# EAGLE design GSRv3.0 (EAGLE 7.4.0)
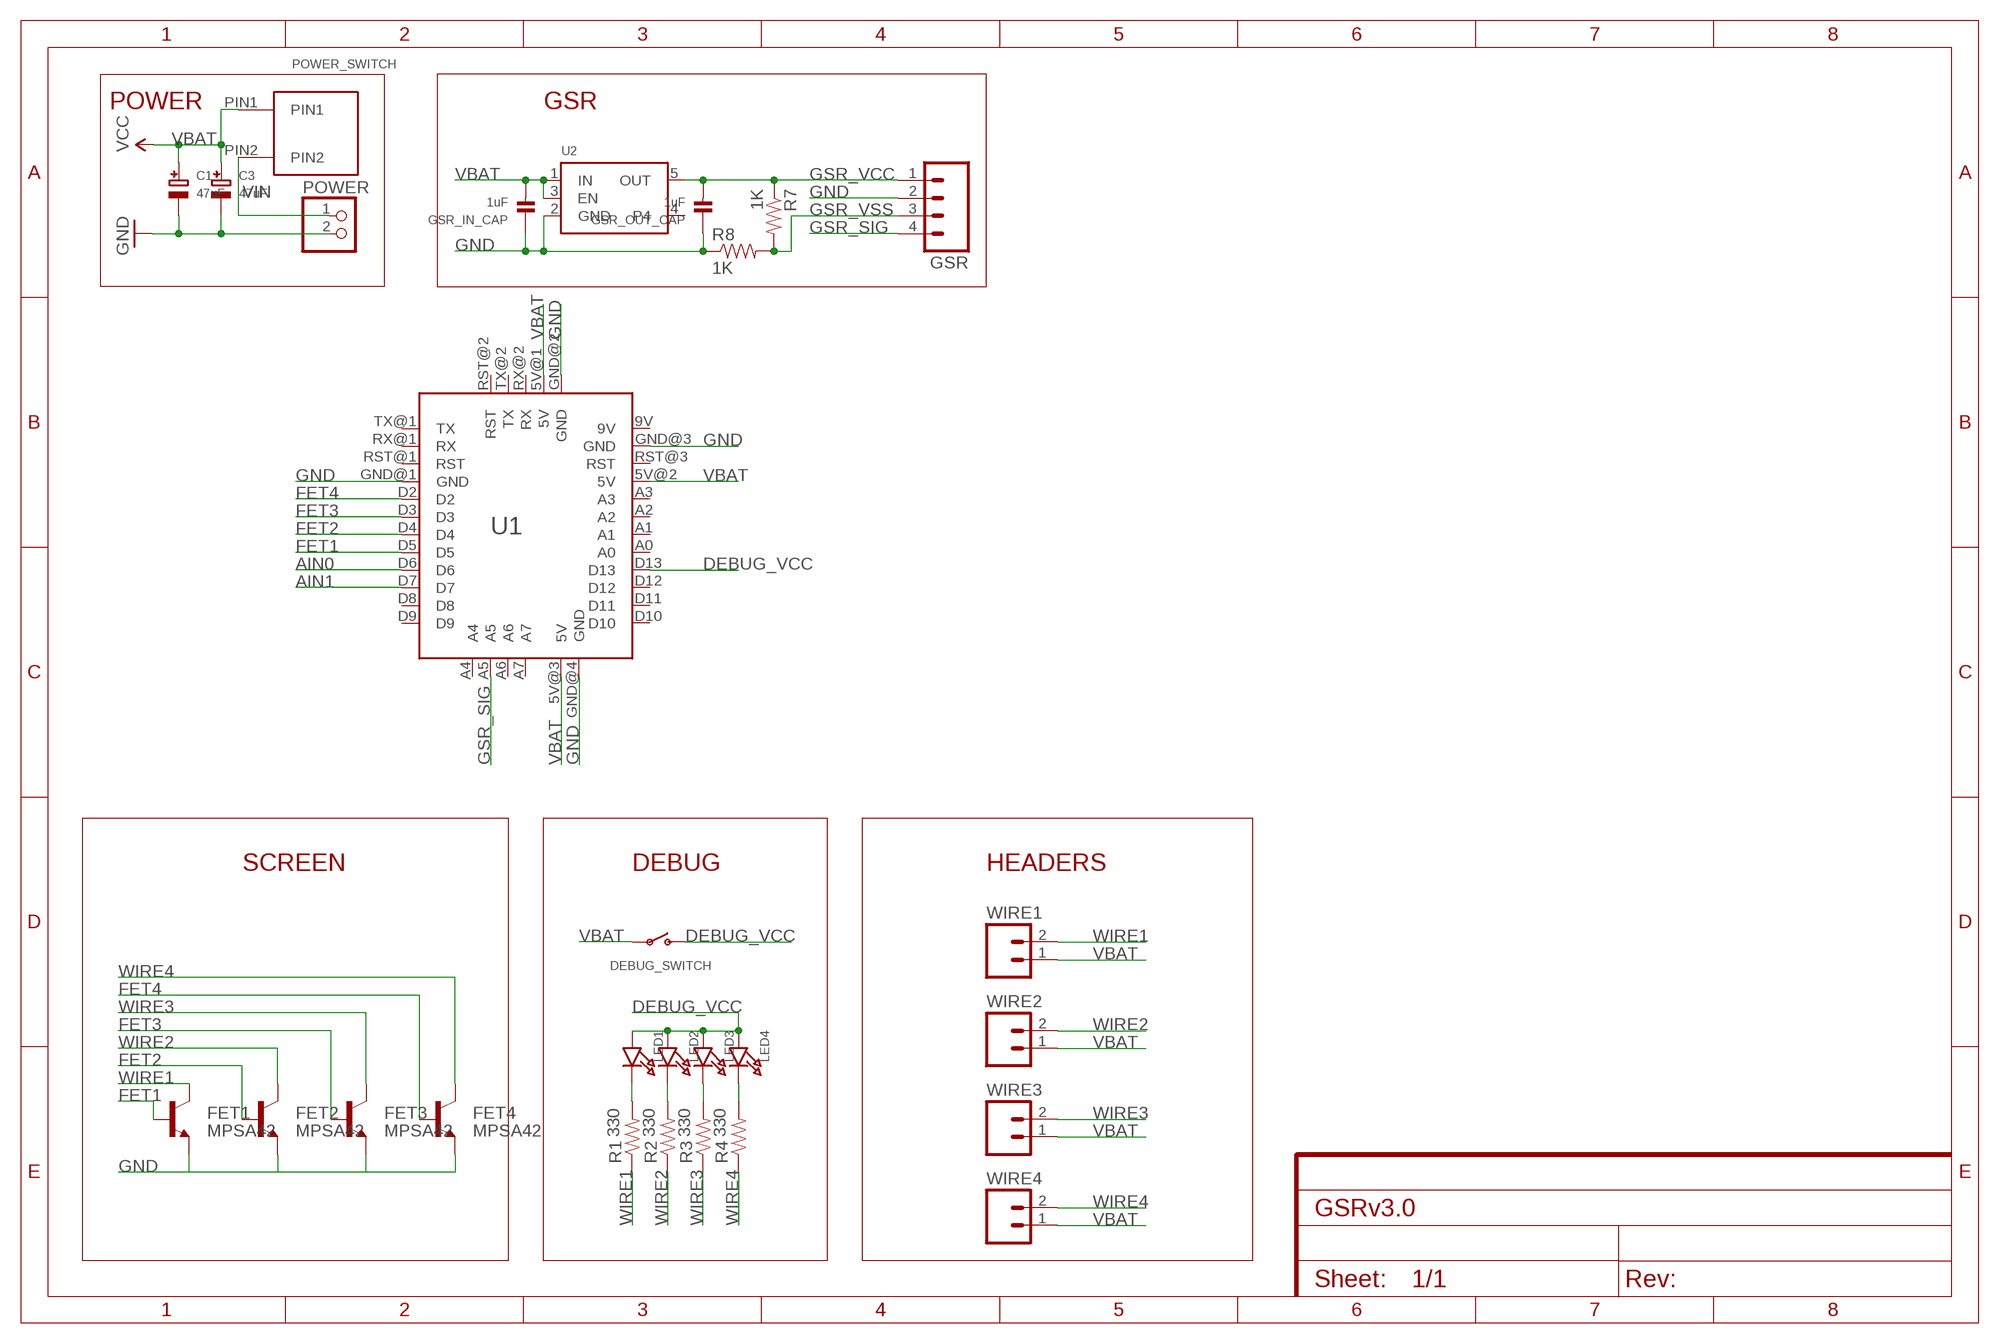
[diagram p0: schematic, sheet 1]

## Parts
C1  47uF  CAP_TANTALUMB/3528_WAVE  [EIA3528-21/B-W]
C3  47uF  CAP_TANTALUMB/3528_WAVE  [EIA3528-21/B-W]
DEBUG_SWITCH  SWITCH_SPST  [SPST_SMT_19192]
FET1  MPSA42  TRANSISTOR_NPNMPSA42  [SOT23-3]
FET2  MPSA42  TRANSISTOR_NPNMPSA42  [SOT23-3]
FET3  MPSA42  TRANSISTOR_NPNMPSA42  [SOT23-3]
FET4  MPSA42  TRANSISTOR_NPNMPSA42  [SOT23-3]
GSR  M04PTH  [1X04]
GSR_IN_CAP  1uF  CAP_CERAMIC0603  [0603]
GSR_OUT_CAP  1uF  CAP_CERAMIC0603  [0603]
LED1  LED0603_NOOUTLINE  [CHIPLED_0603_NOOUTLINE]
LED2  LED0603_NOOUTLINE  [CHIPLED_0603_NOOUTLINE]
LED3  LED0603_NOOUTLINE  [CHIPLED_0603_NOOUTLINE]
LED4  LED0603_NOOUTLINE  [CHIPLED_0603_NOOUTLINE]
POWER  JST_2PIN  [JSTPH2]
POWER_SWITCH  PUSH_BUTTON  [PUSH_BUTTON]
R1  330  RESISTOR0603-RES  [0603-RES]
R2  330  RESISTOR0603-RES  [0603-RES]
R3  330  RESISTOR0603-RES  [0603-RES]
R4  330  RESISTOR0603-RES  [0603-RES]
R7  1K  0OHM-1/10W-5%(0603)  [0603]
R8  1K  0OHM-1/10W-5%(0603)  [0603]
U1  ARDUINO_MINI  [ARDUINO_MINI]
U2  VREG_SOT23-5  [SOT23-5]
WIRE1  M02PTH  [1X02]
WIRE2  M02PTH  [1X02]
WIRE3  M02PTH  [1X02]
WIRE4  M02PTH  [1X02]

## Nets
AIN0: U1.D6
AIN1: U1.D7
DEBUG_VCC: DEBUG_SWITCH.C(S) LED1.A LED2.A LED3.A LED4.A U1.D13
FET1: FET1.1(B) U1.D5
FET2: FET2.1(B) U1.D4
FET3: FET3.1(B) U1.D3
FET4: FET4.1(B) U1.D2
GND: C1.- C3.- FET1.2(E) FET2.2(E) FET3.2(E) FET4.2(E) GSR.2 GSR_IN_CAP.1 GSR_OUT_CAP.1 POWER.2 R8.1 U1.GND@1(GND) U1.GND@2(GND) U1.GND@3(GND) U1.GND@4(GND) U2.2(GND)
GSR_SIG: GSR.4 U1.A5
GSR_VCC: GSR.1 GSR_OUT_CAP.2 R7.1 U2.5(OUT)
GSR_VSS: GSR.3 R7.2 R8.2
N$1: LED1.C R1.2
N$2: LED2.C R2.2
N$3: LED3.C R3.2
N$4: LED4.C R4.2
VBAT: C1.+ C3.+ DEBUG_SWITCH.B(P) GSR_IN_CAP.2 POWER_SWITCH.PIN1 U1.5V@1(5V) U1.5V@2(5V) U1.5V@3(5V) U2.1(IN) U2.3(EN) WIRE1.1 WIRE2.1 WIRE3.1 WIRE4.1 ; supply symbol labelled VCC
VIN: POWER.1 POWER_SWITCH.PIN2
WIRE1: FET1.3(C) R1.1 WIRE1.2
WIRE2: FET2.3(C) R2.1 WIRE2.2
WIRE3: FET3.3(C) R3.1 WIRE3.2
WIRE4: FET4.3(C) R4.1 WIRE4.2
Unconnected: U1.A0 U1.A1 U1.A2 U1.A3 U1.A4 U1.A6 U1.A7 U1.D8 U1.D9 U1.D10 U1.D11 U1.D12 U1.RST@1(RST) U1.RST@2(RST) U1.RST@3(RST) U1.RX@1(RX) U1.RX@2(RX) U1.TX@1(TX) U1.TX@2(TX) U2.4

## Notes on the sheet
- POWER | GSR
- SCREEN | DEBUG | HEADERS

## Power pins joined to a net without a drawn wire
9V: U1.9V

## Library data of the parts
C1 C3 = microbuilder:CAP_TANTALUM: Tantalum Capacitors
DEBUG_SWITCH = microbuilder:SWITCH_SPST: Switch - SPST
FET1-FET4 = SparkFun-DiscreteSemi:TRANSISTOR_NPN: Generic NPN BJT MMBT2222A - TRANS-08049 (SOT-23, 1A 40V) MPSA42 - TRANS-09116 (SOT-23, 500mA 300V) MMBT5088LT1G - TRANS-11160 (SOT-23, 50 mA 30V) BC547 - COM-08928 (TO-92 45V 100mA) (1.Collector 2.Base 3.Emitter) 2N3904 - COM-00521 (TO-92 40V 200mA) (1.Emitter 2.Base 3.Collector) P2N2222A -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; PROD_ID: TRANS-09116
GSR = SparkFun-Connectors:M04: Header 4 Standard 4-pin 0.1" header. Use with straight break away headers (SKU : PRT-00116), right angle break away headers (PRT-00553), swiss pins (PRT-00743), machine pins (PRT-00117), and female headers (PRT-00115). Molex polarized connector foot print use with SKU : PRT-08231 with associated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
GSR_IN_CAP GSR_OUT_CAP = microbuilder:CAP_CERAMIC: Ceramic Capacitors
LED1-LED4 = microbuilder:LED: LED
POWER = microbuilder:JST_2PIN: JST 2-Pin Right-Angle Connector
POWER_SWITCH = myParts:PUSH_BUTTON
R1-R4 = SparkFun-Passives:RESISTOR: Resistor
R7 R8 = SparkFun-Resistors:0OHM-1/10W-5%(0603): RES-08609; PROD_ID: RES-08609; VALUE: 0
U1 = myParts:ARDUINO_MINI: Arduino Mini V5 Footprint
U2 = microbuilder:VREG_SOT23-5: SOT23-5 Fixed Voltage Regulators To better organise some of the SOT23-5 fixed voltage regulators in this library, this new part was created. Part Current Out V Out V In V Dropout Digikey Part No. ADP121 150mA 3.3V 3.4-5.5V 0.09V @ 150mA ADP121-AUJZ33R7CT-ND ADP121 150mA 3.0V 3.1-5.5V 0.09V @ 150mA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
WIRE1-WIRE4 = SparkFun-Connectors:M02: Standard 2-pin 0.1" header. Use with

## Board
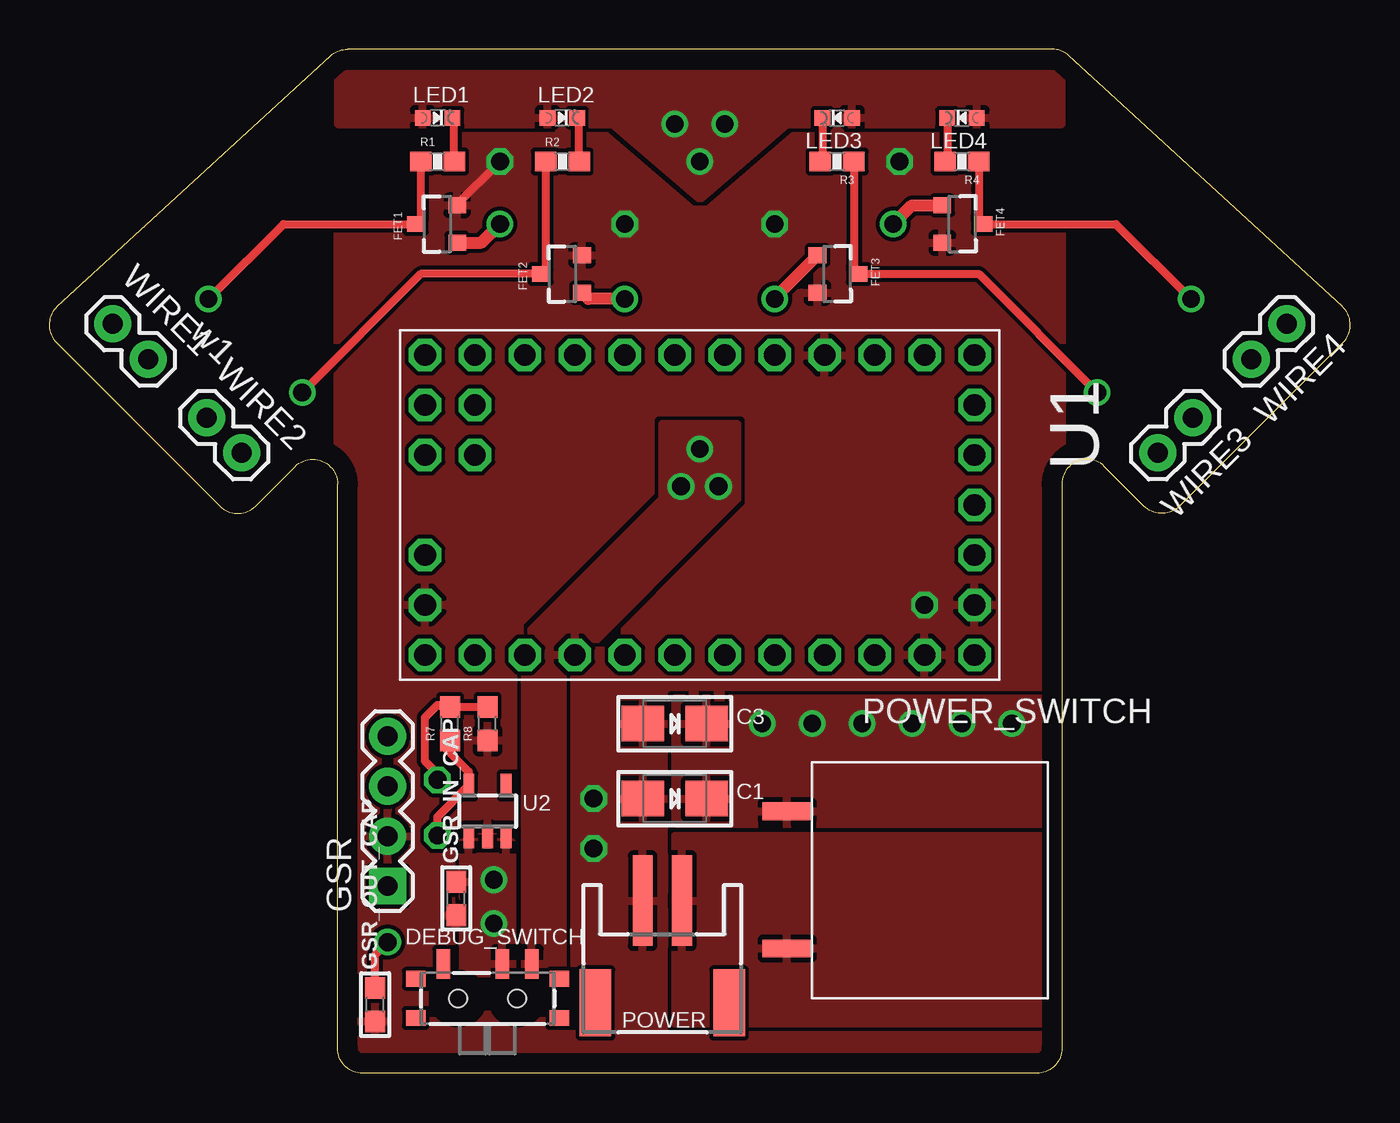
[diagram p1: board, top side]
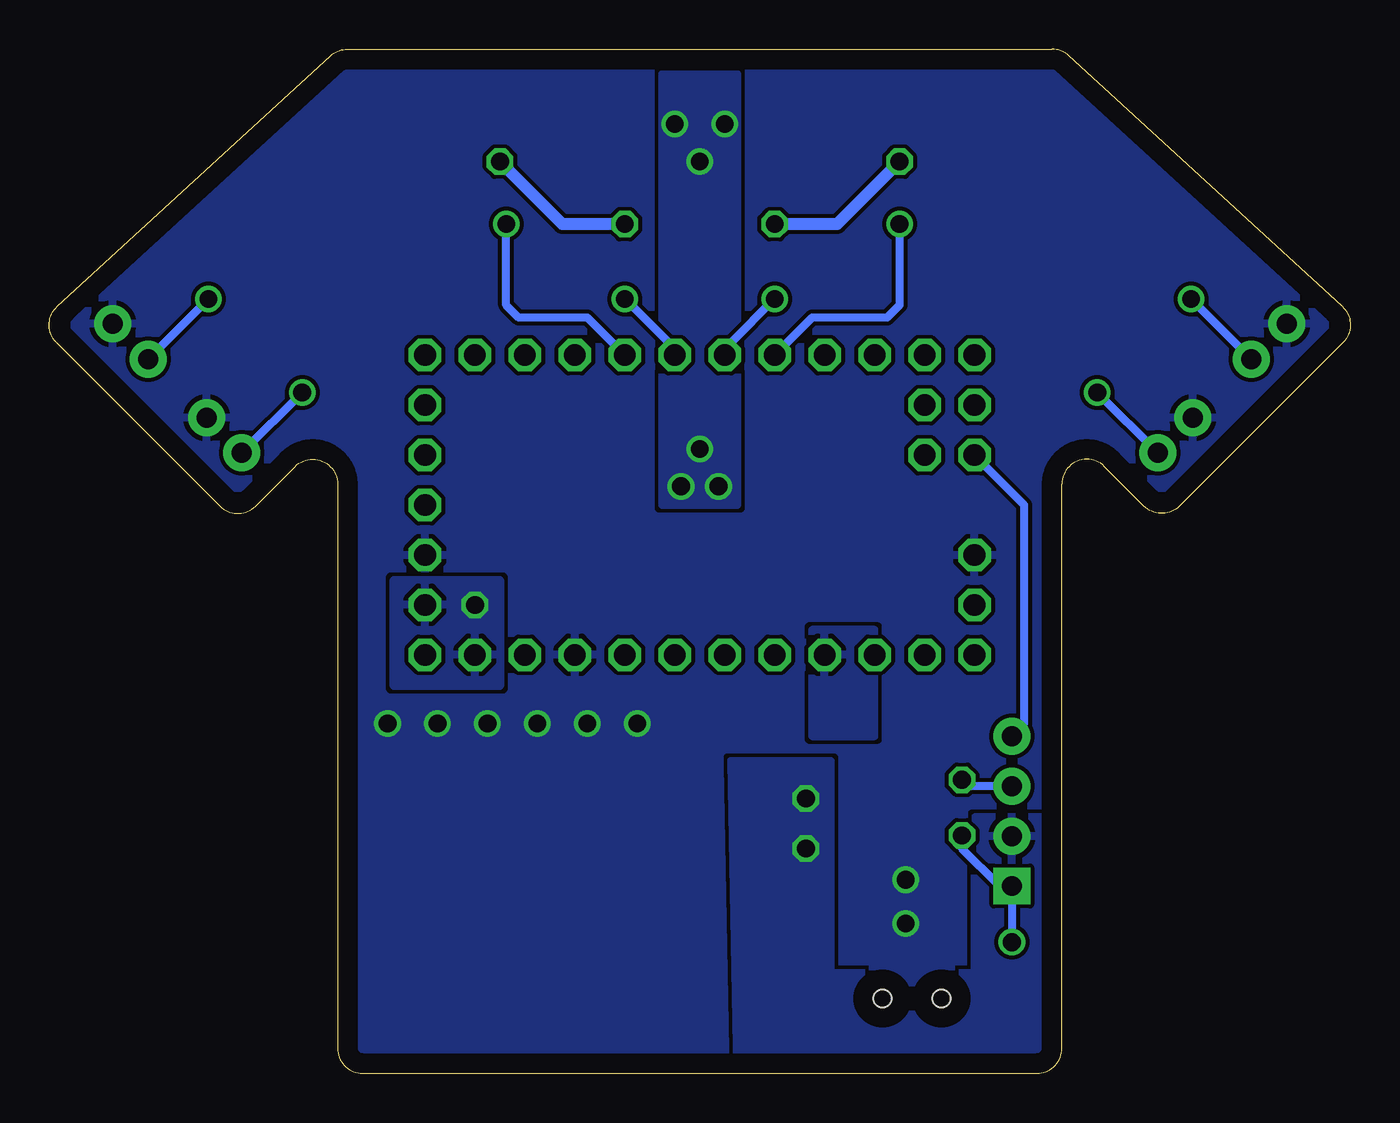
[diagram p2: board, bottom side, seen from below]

Size 66.18 x 52.07 mm. Coordinates in mm from the lower left corner, seen from the top.
Outline: 0.41,39 14.31,51.74 arc-43 15.17,52.07 51.01,52.07 arc-43 51.87,51.74 65.77,39 arc-92 65.81,37.16 57.48,28.84 arc-90 55.69,28.84 53.67,30.85 arc135 51.5,29.95 51.5,1.27 arc-90 50.23,0 15.94,0 arc-90 14.67,1.27 14.67,29.95 arc135 12.51,30.85 10.49,28.84 arc-90 8.7,28.84 0.37,37.16 arc-92 0.41,39
Copper layers (1*16): Top 0.035mm / dielectric 1.5mm / Bottom 0.035mm
Design rules "default": minimum track width 10mil, minimum drill 24mil, track to track 8mil, track to pad 8mil, pad to pad 8mil, via to via 8mil, smd to smd 8mil, copper to edge 40mil, drill to drill 8mil, minimum pad ring 10mil, minimum via ring 8mil, stop-mask expansion 4mil, vias tented up to drill 0mil, thermal gap 10mil

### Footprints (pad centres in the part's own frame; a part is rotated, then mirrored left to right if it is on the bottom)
EIA3528-21/B-W = smd 2.15 x 1.8: + 1.625,0; - -1.625,0
SPST_SMT_19192 = smd 0.7 x 1.5: A -2.25,1.75; B 0.75,1.75; C 2.25,1.75 | smd 1 x 0.8: GND1 -3.65,1; GND2 -3.65,-1; GND3 3.65,1; GND4 3.65,-1 | hole 0.9: -1.5,0; 1.5,0
SOT23-3 = smd 0.8 x 0.9: 1 -0.95,-1; 2 0.95,-1; 3 0,1.1
1X04 = drill 1.016 pad 1.88 square: 1 0,0 | drill 1.016 pad 1.88: 2 2.54,0; 3 5.08,0; 4 7.62,0
0603 = smd 1.1 x 1: 1 -0.85,0; 2 0.85,0
CHIPLED_0603_NOOUTLINE = smd 0.8 x 0.8: A 0,-0.75; C 0,0.75
JSTPH2 = smd 1 x 4.6: 1 -1,-3.7; 2 1,-3.7 | smd 1.6 x 3.4: NC1 -3.4,1.5; NC2 3.4,1.5
PUSH_BUTTON = smd 2.5 x 0.9: PIN1 -13.97,-0.644; PIN2 -13.97,-7.62
0603-RES = smd 1.1 x 1: 1 -0.85,0; 2 0.85,0
ARDUINO_MINI = drill 1.1 octagon: 5V@1 2.54,15.24; 5V@2 7.62,7.62; 5V@3 2.54,-12.7; 9V 7.62,15.24; A0 7.62,-2.54; A1 7.62,0; A2 7.62,2.54; A3 7.62,5.08; A4 -5.08,-12.7; A5 -2.54,-12.7; A6 -5.08,-10.16; A7 -2.54,-10.16; D2 -7.62,5.08; D3 -7.62,2.54; D4 -7.62,0; D5 -7.62,-2.54; D6 -7.62,-5.08; D7 -7.62,-7.62; D8 -7.62,-10.16; D9 -7.62,-12.7; D10 7.62,-12.7; D11 7.62,-10.16; D12 7.62,-7.62; D13 7.62,-5.08; GND@1 -7.62,7.62; GND@2 5.08,15.24; GND@3 7.62,12.7; GND@4 5.08,-12.7; RST@1 -7.62,10.16; RST@2 -5.08,15.24; RST@3 7.62,10.16; RX@1 -7.62,12.7; RX@2 0,15.24; TX@1 -7.62,15.24; TX@2 -2.54,15.24
SOT23-5 = smd 0.55 x 1.2: 1 -0.95,-1.3; 2 0,-1.3; 3 0.95,-1.3; 4 0.95,1.3; 5 -0.95,1.3
1X02 = drill 1.016 pad 1.88: 1 0,0; 2 2.54,0

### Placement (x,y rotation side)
C1  31.82,13.97 0 top
C3  31.82,17.78 0 top
DEBUG_SWITCH  22.29,3.81 0 top
FET1  19.75,43.18 90 top
FET2  26.1,40.64 90 top
FET3  40.07,40.64 270 top
FET4  46.42,43.18 270 top
GSR  17.21,9.53 90 top
GSR_IN_CAP  20.71,8.89 90 top
GSR_OUT_CAP  16.58,3.49 90 top
LED1  19.75,48.58 270 top
LED2  26.1,48.58 270 top
LED3  40.07,48.58 90 top
LED4  46.42,48.58 90 top
POWER  31.18,5.08 180 top
POWER_SWITCH  51.5,13.97 0 top
R1  19.75,46.35 0 top
R2  26.1,46.35 0 top
R3  40.07,46.35 180 top
R4  46.42,46.35 180 top
R7  20.39,17.78 90 top
R8  22.29,17.78 90 top
U1  31.82,28.89 270 top
U2  22.29,13.34 0 top
WIRE1  3.24,38.1 315 top
WIRE2  8.01,33.34 315 top
WIRE3  58.17,33.34 225 top
WIRE4  62.93,38.1 225 top

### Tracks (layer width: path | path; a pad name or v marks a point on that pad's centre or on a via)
DEBUG_VCC  (via drill 0.9)
  other vias: 33.09,31.75 32.14,29.84 34.04,29.84 33.09,46.35 31.82,48.26 34.36,48.26
  pour Bottom: 34.99,28.89 34.99,50.8 31.18,50.8 31.18,28.89
  pour Top: 33.09,44.45 37.53,48.26 51.5,48.26 51.5,50.8 14.67,50.8 14.67,48.26 28.64,48.26
  pour Top: 24.2,5.08 24.2,21.59 26.1,21.59 26.1,5.08
  pour Top: 31.18,33.02 34.99,33.02 34.99,29.21 26.1,20.32 23.56,20.32 23.56,21.59 31.18,29.21
  pour Bottom: 24.2,22.54 27.37,22.54 27.37,17.14 24.2,17.14
FET1  (via drill 0.9)
  Top 0.61: FET1.1 21.98,42.23 v22.93,43.18
  Bottom 0.406: v22.93,43.18 22.93,39.05 23.56,38.42 27.37,38.42 U1.D5
FET2  (via drill 0.9)
  Top 0.61: v29.28,39.37 27.42,39.37 FET2.1
  Bottom 0.406: U1.D4 31.5,36.51 31.5,37.15 v29.28,39.37
FET3  (via drill 0.9)
  Top 0.406: v36.9,39.37 36.9,39.41
  Top 0.61: 36.9,39.41 FET3.1
  Bottom 0.406: v36.9,39.37 34.36,36.83 U1.D3
FET4  (via drill 0.9)
  Top 0.406: FET4.1
  Top 0.61: v42.93,43.18 43.88,44.13 FET4.1
  Bottom 0.406: U1.D2 38.8,38.42 42.3,38.42 42.93,39.05 v42.93,43.18
GND  (via drill 0.9)
  Top 0.406: FET1.2 20.75,44.18 v22.93,46.35
  Bottom 0.61: v29.28,43.18 26.1,43.18 v22.93,46.35 | v36.9,43.18 40.07,43.18 v43.25,46.35
  other vias: 27.69,11.43 27.69,13.97 44.52,23.81
  pour Top (rank 3): 14.67,58.42 51.5,58.42 51.5,-6.35 14.67,-6.35
  pour Bottom: 14.67,13.02 19.12,13.02 19.12,5.08 26.42,5.08 26.42,15.88 31.5,15.88 31.18,0 14.67,0
  pour Bottom: 48.65,25.08 43.25,25.08 43.25,19.68 48.65,19.68
GSR_SIG
  Bottom 0.406: GSR.4 16.58,17.78 16.58,28.89 U1.A5
GSR_VCC  (via drill 0.9)
  Top 0.406: R7.1 20.07,16.61 21.34,15.34 U2.5 19.75,13.05 v19.75,12.09 | GSR_OUT_CAP.2 16.58,6.03 v17.21,6.67
  Bottom 0.406: v19.75,12.09 19.75,11.43 17.85,9.53 GSR.1 v17.21,6.67
GSR_VSS  (via drill 0.9)
  Top 0.406: 19.97,18.63 R7.2 | R7.2 R8.2 | v19.75,14.92 19.75,15.24 19.12,15.88 19.12,18.1 19.75,18.73 20.29,18.73 R7.2
  Bottom 0.406: GSR.3 19.44,14.61 v19.75,14.92
N$1
  Top 0.406: R1.2 20.6,48.48 LED1.C
N$2
  Top 0.406: R2.2 26.95,48.48 LED2.C
N$3
  Top 0.406: LED3.C 39.32,46.45 R3.2
N$4
  Top 0.406: LED4.C 45.67,46.45 R4.2
VBAT  (via drill 0.9)
  other vias: 22.61,9.84 22.61,7.62 41.34,17.78 38.8,17.78 36.26,17.78 43.88,17.78 46.42,17.78 48.96,17.78
  pour Bottom (rank 2): -6.92,55.88 76.9,55.88 76.9,-2.54 -6.92,-2.54
  pour Top: 51.5,19.05 31.82,19.05 31.82,12.7 51.5,12.7
  pour Top: 23.56,11.75 21.02,11.75 21.02,5.08 23.56,5.08
VIN
  pour Top: 51.5,12.07 31.82,12.07 31.82,2.54 51.5,2.54
WIRE1  (via drill 0.9)
  Top 0.406: R1.1 18.9,43.43 FET1.3 11.92,43.18 v8.11,39.37
  Bottom 0.406: v8.11,39.37 WIRE1.2
WIRE2  (via drill 0.9)
  Top 0.406: R2.1 25.25,40.89 FET2.3 18.9,40.64 v12.87,34.61
  Bottom 0.406: v12.87,34.61 WIRE2.2
WIRE3  (via drill 0.9)
  Top 0.406: R3.1 40.92,40.89 FET3.3 47.28,40.64 v53.31,34.61
  Bottom 0.406: v53.31,34.61 WIRE3.2
WIRE4  (via drill 0.9)
  Top 0.406: R4.1 47.27,43.43 FET4.3 54.26,43.18 v58.07,39.37
  Bottom 0.406: v58.07,39.37 WIRE4.2

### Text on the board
tSilk: w1

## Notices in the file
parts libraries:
SparkFun-Aesthetics: Licensing: Creative Commons ShareAlike 4.0 International - https://creativecommons.org/licenses/by-sa/4.0
microbuilder: This work is placed in the public domain, and may be freely used for commercial and non-commercial work with the following conditions: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
